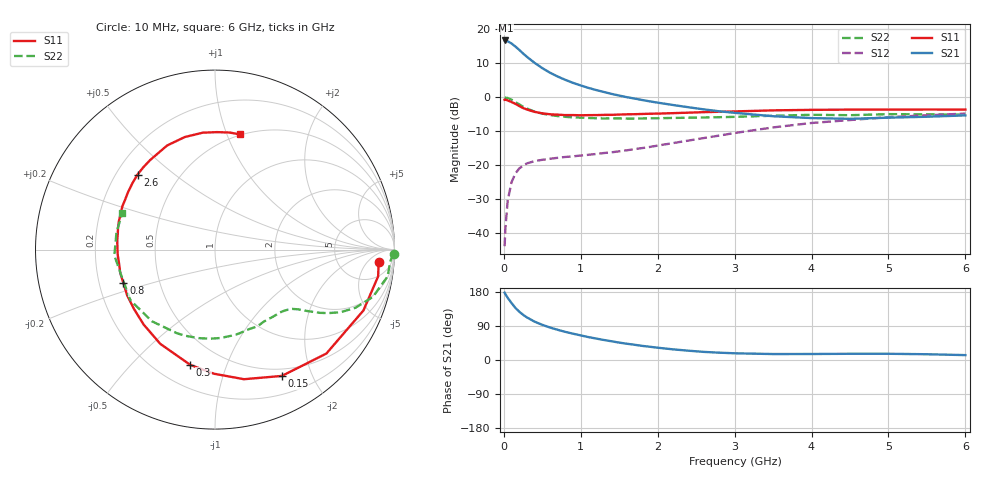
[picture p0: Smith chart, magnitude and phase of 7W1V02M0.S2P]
! Infineon Technologies  Discrete & RF Semiconductors
! BFS17W
! Si NPN RF Bipolar Junction Transistor in SOT323
! VCE = 1 V  IC = 2 mA
! Common Emitter S-Parameters:  August  1999
# GHz  S  MA  R  50
!  f  S11  S21  S12  S22
! GHz  MAG  ANG  MAG  ANG  MAG  ANG  MAG  ANG
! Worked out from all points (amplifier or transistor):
!   36 points, 10 MHz to 6 GHz, reference 50 ohm
!   highest |S21| = 16.8 dB at 20 MHz (marker M1)
!   |S21| within 3 dB of that: start of sweep to 210.5 MHz
!   unconditionally stable (mu >= 1): 761.9 MHz to end of sweep
!   at 250 MHz: K = 0.38, MSG = 16.6 dB, |S12| = -20.2 dB
!   at 1.4 GHz: K = 1.39, MAG = 4.9 dB, |S12| = -16.3 dB
!   at 6 GHz: K = 1.13, MAG = -2.5 dB, |S12| = -4.9 dB
!   S11 on the Smith chart (normalised r, x): 10 MHz: 13, -11; 150 MHz: 0.41, -1.58; 300 MHz: 0.33, -0.75; 800 MHz: 0.30, -0.16; 2.6 GHz: 0.29, +0.38; 6 GHz: 0.49, +1.11
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0.01  0.9143 -4.4  6.846 177.6  0.0063 84.6  0.9968 -1.3
0.02  0.9211 -9.3  6.881 173.8  0.0114 87.9  0.9801 -3.5
0.05  0.8938 -22.3  6.689 164.3  0.0297 78.5  0.9727 -8.9
0.1  0.8488 -43.0  6.207 150.2  0.0555 66.3  0.9182 -16.7
0.15  0.7964 -62.1  5.6 137.6  0.0746 56.9  0.8469 -22.5
0.2  0.7399 -77.4  4.998 127.6  0.0884 50.6  0.7821 -26.5
0.25  0.6915 -90.5  4.423 119.3  0.0975 44.9  0.7231 -29.3
0.3  0.6569 -102.1  3.947 112.4  0.1052 41.4  0.6799 -31.2
0.4  0.6073 -120.1  3.21 101.2  0.1136 36.9  0.6117 -33.9
0.5  0.5765 -133.6  2.683 92.8  0.1188 34.9  0.572 -35.6
0.6  0.5594 -144.0  2.298 85.7  0.1231 33.9  0.5442 -37.4
0.8  0.5434 -159.9  1.801 74.2  0.1309 34.3  0.5125 -41.9
1.1  0.5427 -176.7  1.371 60.4  0.1409 37.3  0.4931 -49.8
1.3  0.5473 174.4  1.193 52.8  0.1496 39.9  0.4848 -56.1
1.6  0.5582 163.7  0.999 42.9  0.1642 44.1  0.4829 -65.7
2.2  0.5809 146.4  0.766 28.1  0.2099 50.6  0.4936 -86.4
2.6  0.601 135.9  0.66 21.4  0.249 52.1  0.5015 -100.5
3.5  0.6385 114.7  0.523 15.7  0.3575 48.7  0.5321 -131.4
4  0.6494 105.0  0.491 15.8  0.4157 43.4  0.5492 -149.0
4.5  0.655 95.9  0.479 16.4  0.4593 37.6  0.5415 -164.3
5.5  0.6574 82.8  0.514 15.2  0.5396 26.8  0.5573 169.9
6  0.6561 77.8  0.538 12.9  0.5721 21.5  0.5544 158.6
